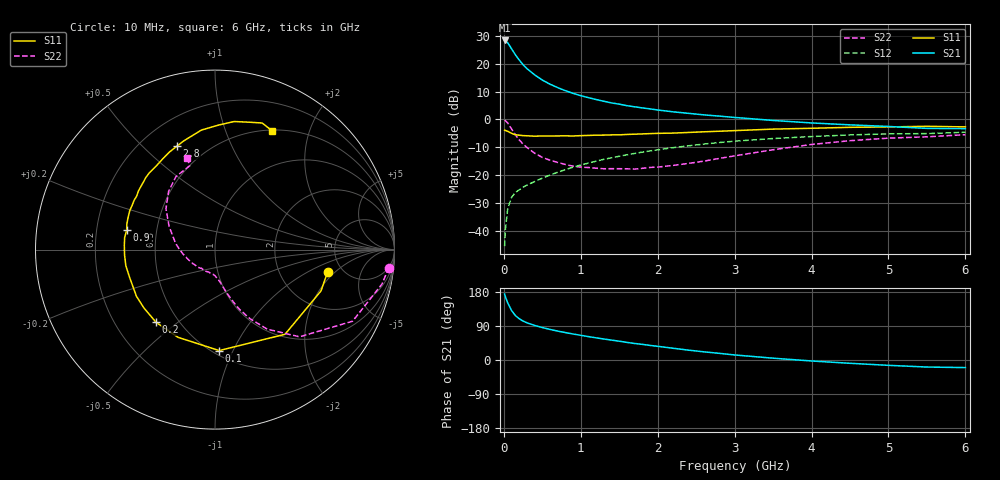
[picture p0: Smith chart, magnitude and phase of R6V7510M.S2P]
! SIEMENS Small Signal Semiconductors
! BFR193
! Si NPN RF Bipolar Junction Transistor in SOT23
! VCE = 0.75 V  IC = 10 mA
! Common Emitter S-Parameters:  May  1996
# GHz  S  MA  R  50
!  f  S11  S21  S12  S22
! GHz  MAG  ANG  MAG  ANG  MAG  ANG  MAG  ANG
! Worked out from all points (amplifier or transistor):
!   36 points, 10 MHz to 6 GHz, reference 50 ohm
!   highest |S21| = 28.4 dB at 10 MHz (marker M1)
!   |S21| within 3 dB of that: start of sweep to 100.4 MHz
!   unconditionally stable (mu >= 1): 678.8 MHz to 2.325 GHz
!   at 250 MHz: K = 0.66, MSG = 22.0 dB, |S12| = -24.3 dB
!   at 1.4 GHz: K = 1.05, MAG = 8.4 dB, |S12| = -13.8 dB
!   at 6 GHz: K = 0.98, MSG = 0.6 dB, |S12| = -4.6 dB
!   S11 on the Smith chart (normalised r, x): 10 MHz: 3.86, -1.60; 100 MHz: 0.54, -0.89; 200 MHz: 0.38, -0.42; 900 MHz: 0.33, +0.10; 2.8 GHz: 0.35, +0.64; 6 GHz: 0.51, +1.46
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0.01  0.64 -11.0  26.2 173.9  0.0053 84.9  0.9732 -5.9
0.02  0.6339 -21.3  25.95 167.4  0.0106 79.7  0.9505 -11.6
0.05  0.6122 -50.4  23.87 150.8  0.0247 69.5  0.8641 -27.5
0.1  0.563 -87.6  18.58 130.8  0.0398 57.4  0.6768 -45.9
0.15  0.5304 -112.9  14.52 117.3  0.0489 52.2  0.5303 -56.7
0.2  0.5215 -129.0  11.67 108.9  0.0544 50.7  0.4303 -63.2
0.25  0.5124 -140.6  9.621 102.8  0.0607 50.7  0.3614 -67.6
0.3  0.5091 -149.3  8.195 98.2  0.0661 51.8  0.3146 -70.4
0.4  0.5004 -162.1  6.323 91.2  0.0767 54.2  0.2481 -75.0
0.5  0.5048 -169.8  5.098 85.6  0.0882 56.3  0.208 -78.3
0.6  0.5048 -176.7  4.297 80.7  0.1002 57.3  0.1852 -80.8
0.7  0.5057 177.2  3.73 76.2  0.1125 58.2  0.1691 -83.6
0.9  0.5041 167.6  2.941 68.6  0.1391 59.0  0.1446 -90.4
1.1  0.5165 159.4  2.461 61.7  0.1647 58.5  0.1369 -97.5
1.3  0.5232 152.2  2.118 55.4  0.192 57.2  0.1302 -105.5
1.6  0.5377 142.3  1.767 46.5  0.2317 54.6  0.1298 -120.1
2.2  0.5686 125.5  1.37 31.0  0.3113 47.2  0.1495 -150.9
2.8  0.6137 110.3  1.148 17.6  0.3846 38.5  0.1994 179.1
3.5  0.6703 96.5  0.959 4.8  0.4537 27.3  0.2857 153.4
4.5  0.7215 81.5  0.799 -8.7  0.5268 12.8  0.4153 128.5
5.5  0.7526 69.6  0.691 -18.6  0.5566 -1.3  0.4876 106.8
6  0.7348 64.5  0.684 -20.0  0.5898 -5.4  0.5318 107.0
